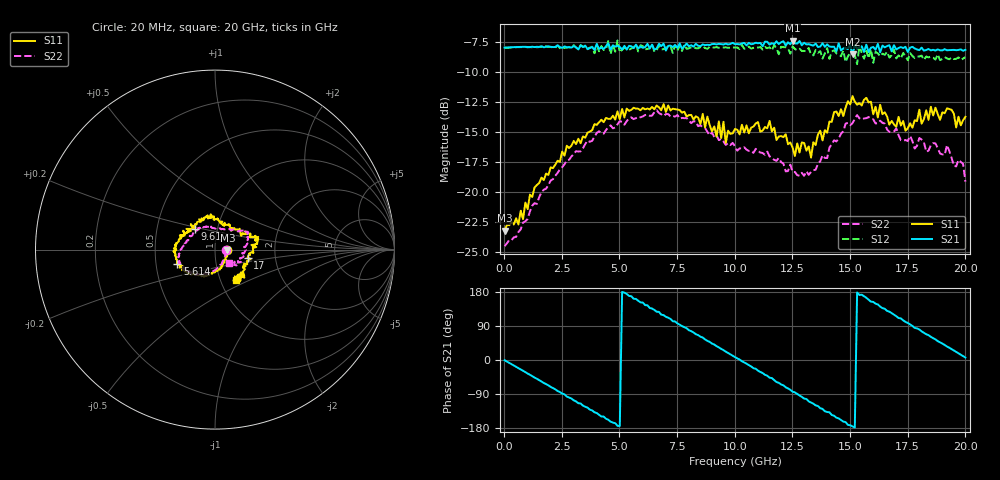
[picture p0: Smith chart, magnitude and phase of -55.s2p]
!Agilent Technologies,N5230A,US43500223,A.07.50.48
!Agilent N5230A: A.07.50.48
!Date: Thursday, October 08, 2015 19:25:47
!Correction: S11(Full 2 Port(1,2))
!S21(Full 2 Port(1,2))
!S12(Full 2 Port(1,2))
!S22(Full 2 Port(1,2))
!S2P File: Measurements: S11, S21, S12, S22:
# Hz S  RI  R 50
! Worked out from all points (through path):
!   201 points, 20 MHz to 20 GHz, reference 50 ohm
!   highest |S21| = -7.41 dB at 12.51 GHz (marker M1); lowest = -8.5 dB at 15.1 GHz (marker M2)
!   group delay of S21, straight-line fit = 99.1 ps
!   lowest |S11| = -23.2 dB at 20 MHz (marker M3), VSWR 1.15, Z = 57.4 - j0.208 ohm
!   |S11| at or under -10 dB: start of sweep to end of sweep
!   |S22| runs from -24.5 to -13.2 dB; largest |S21 - S12| = 0.066
!   S11 on the Smith chart (normalised r, x): 20 MHz: 1.15, -0.00; 5.614 GHz: 0.65, -0.11; 9.61 GHz: 0.78, +0.18; 17 GHz: 1.44, -0.13; 20 GHz: 1.19, -0.42
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2e7  0.069 -0.00181  0.3987 -0.00458  0.3985 -0.00569  0.0595 -0.00287
1.8182e9  0.014 -0.1186  0.1787 -0.3604  0.1732 -0.3658  0.015 -0.1021
3.4166e9  -0.0921 -0.1434  -0.2025 -0.3467  -0.2198 -0.3362  -0.0694 -0.1353
4.9151e9  -0.184 -0.1143  -0.4038 -0.0451  -0.4258 -0.0358  -0.1496 -0.1192
5.6144e9  -0.2096 -0.0798  -0.3764 0.126  -0.3723 0.1425  -0.172 -0.1043
6.7133e9  -0.2244 -0.0175  -0.2487 0.3305  -0.2289 0.3375  -0.2006 -0.0722
7.9121e9  -0.2006 0.0471  0.0447 0.4122  0.0735 0.3872  -0.2016 -0.0247
9.4106e9  -0.122 0.1151  0.3598 0.2019  0.3591 0.1737  -0.1599 0.046
9.5105e9  -0.135 0.1421  0.3695 0.1803  0.3703 0.1501  -0.1531 0.054
9.6104e9  -0.1134 0.1129  0.3841 0.1555  0.3794 0.127  -0.1485 0.0514
1.001e10  -0.1002 0.1532  0.4088 0.0559  0.3983 0.0284  -0.1358 0.074
1.14086e10  -0.0298 0.1817  0.3159 -0.2797  0.275 -0.2858  -0.0724 0.1283
1.25075e10  0.0275 0.1509  0.0473 -0.4234  0.0247 -0.4027  -0.017 0.1201
1.34066e10  0.1078 0.1198  -0.1726 -0.368  -0.174 -0.3267  0.0452 0.1148
1.45055e10  0.1938 0.0735  -0.3741 -0.1818  -0.3375 -0.1603  0.1328 0.1012
1.51049e10  0.2407 0.0705  -0.3724 -0.032  -0.3755 0.0184  0.1662 0.0991
1.57043e10  0.2392 0.0597  -0.3947 0.1117  -0.3725 0.1053  0.1823 0.0893
1.67033e10  0.1894 -0.0226  -0.2488 0.3238  -0.1985 0.3032  0.172 0.0455
1.7003e10  0.1816 -0.0441  -0.1703 0.3528  -0.1212 0.3387  0.1809 0.0347
1.84016e10  0.1441 -0.1383  0.1635 0.3582  0.1757 0.318  0.141 -0.0472
1.92008e10  0.1418 -0.172  0.3165 0.2261  0.3104 0.1818  0.135 -0.0801
2e10  0.1176 -0.1687  0.388 0.0442  0.3641 0.00903  0.0805 -0.0757
